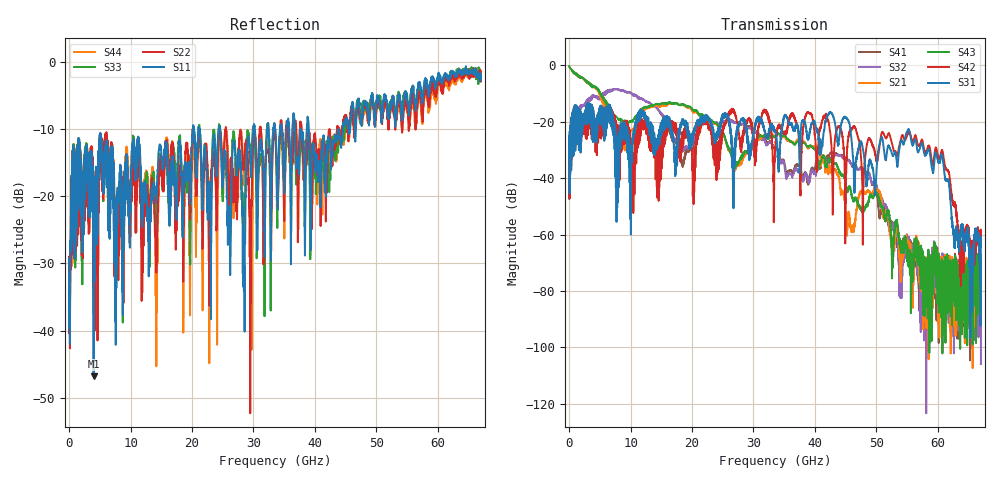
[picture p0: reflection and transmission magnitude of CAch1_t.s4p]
!Agilent Technologies,N5247A,US51170199,A.09.90.13
!Agilent N5247A: A.09.90.13
!Date: Wednesday, October 17, 2018 15:27:01
!Correction: S11(Full 4 Port(1,2,3,4))
!S12(Full 4 Port(1,2,3,4))
!S13(Full 4 Port(1,2,3,4))
!S14(Full 4 Port(1,2,3,4))
!S21(Full 4 Port(1,2,3,4))
!S22(Full 4 Port(1,2,3,4))
!S23(Full 4 Port(1,2,3,4))
!S24(Full 4 Port(1,2,3,4))
!S31(Full 4 Port(1,2,3,4))
!S32(Full 4 Port(1,2,3,4))
!S33(Full 4 Port(1,2,3,4))
!S34(Full 4 Port(1,2,3,4))
!S41(Full 4 Port(1,2,3,4))
!S42(Full 4 Port(1,2,3,4))
!S43(Full 4 Port(1,2,3,4))
!S44(Full 4 Port(1,2,3,4))
!S4P File: Measurements: <S11,S12,S13,S14>,
!<S21,S22,S23,S24>,
!<S31,S32,S33,S34>,
!<S41,S42,S43,S44>:
# Hz S  dB  R 50
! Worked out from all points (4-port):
!   6701 points, 10 MHz to 67 GHz, reference 50 ohm
!   strongest paths, dB at 10 MHz, 16.76 GHz, 33.51 GHz, 50.25 GHz, 67 GHz:
!     S31: -32.9, -25.1, -23.7, -31.2, -64.4
!     S42: -33.0, -20.8, -30.1, -32.5, -58.3
!     S43: -0.3, -13.6, -25.2, -45.9, -72.7
!     S21: -0.3, -13.7, -25.0, -44.4, -80.3
!     S32: -47.1, -24.4, -29.4, -44.8, -105.9
!     S41: -47.2, -25.9, -29.3, -48.2, -77.7
!   lowest |S11| = -46.8 dB at 3.989 GHz (marker M1), VSWR 1.01, Z = 49.9 - j0.438 ohm
!   |S11| at or under -10 dB: start of sweep to 20.18 GHz; 24.53 GHz to 29.98 GHz (5.455 GHz wide, 20 % of centre); 39.02 GHz to 43.83 GHz (4.815 GHz wide, 11.6 % of centre)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
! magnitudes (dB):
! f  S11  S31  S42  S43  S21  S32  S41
! 10 MHz  -30.2  -32.9  -33.0  -0.3  -0.3  -47.1  -47.2
! 3.989 GHz  -46.8  -26.4  -24.6  -7.3  -7.4  -10.8  -10.7
! 39.44 GHz  -18.5  -20.8  -17.7  -28.7  -28.7  -37.4  -36.5
! 47.81 GHz  -6.9  -29.8  -55.0  -52.6  -44.7  -37.9  -36.9
! 55.17 GHz  -6.5  -22.8  -24.0  -66.9  -64.0  -61.2  -61.8
! 63.87 GHz  -1.4  -57.5  -63.4  -80.4  -90.9  -70.9  -81.0
! 67 GHz  -2.4  -64.4  -58.3  -72.7  -80.3  -105.9  -77.7
